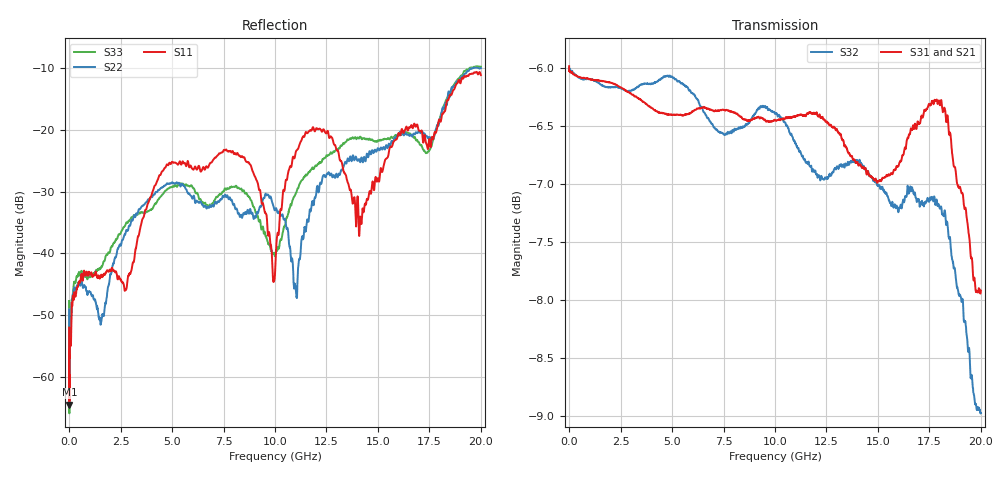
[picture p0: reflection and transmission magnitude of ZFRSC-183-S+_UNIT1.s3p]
!Mini-Circuits Laboratory
!S-Parameters
!Model: ZFRSC-183-S+
!Run/Lot/Date Code: F89730/NA/1038
!Fixture/SN/Due: NOT REQUIRED
!Connection: PORT 1 - SUM, PORT 2 - 1, PORT 3 - 2.
!Tested By: JIAN CHEN
!UNIT S/N: 1
!Agilent Technologies,N5230A,MY45001447,A.07.50.63
!Agilent N5230A: A.07.50.63
!Date: Wednesday, April 06, 2011 14:43:44
!Correction: S11(Full 3 Port(1,2,3))
!S12(Full 3 Port(1,2,3))
!S13(Full 3 Port(1,2,3))
!S21(Full 3 Port(1,2,3))
!S22(Full 3 Port(1,2,3))
!S23(Full 3 Port(1,2,3))
!S31(Full 3 Port(1,2,3))
!S32(Full 3 Port(1,2,3))
!S33(Full 3 Port(1,2,3))
!S3P File: Measurements: <S11,S12,S13>,
!<S21,S22,S23>,
!<S31,S32,S33>:
# Hz S  dB  R 50
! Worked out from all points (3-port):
!   2097 points, 300 kHz to 20 GHz, reference 50 ohm
!   strongest paths, dB at 300 kHz, 4.28 GHz, 9.52 GHz, 14.76 GHz, 20 GHz:
!     S31: -6.0, -6.4, -6.4, -6.9, -7.9
!     S21: -6.0, -6.3, -6.4, -7.0, -8.1
!     S32: -6.0, -6.1, -6.3, -7.0, -9.0
!   lowest |S11| = -64.6 dB at 13 MHz (marker M1), VSWR 1.00, Z = 50 + j0.0587 ohm
!   |S11| at or under -10 dB: start of sweep to end of sweep
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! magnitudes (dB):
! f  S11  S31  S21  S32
! 300 kHz  -52.1  -6.0  -6.0  -6.0
! 13 MHz  -64.6  -6.0  -6.0  -6.0
! 410 MHz  -45.5  -6.1  -6.1  -6.1
! 4.81 GHz  -25.7  -6.4  -6.4  -6.1
! 8.47 GHz  -24.5  -6.4  -6.4  -6.5
! 10.01 GHz  -42.8  -6.4  -6.4  -6.4
! 11 GHz  -23.7  -6.4  -6.4  -6.7
! 11.55 GHz  -20.6  -6.4  -6.4  -6.8
! 14.15 GHz  -34.2  -6.8  -7.0  -6.8
! 20 GHz  -11.1  -7.9  -8.1  -9.0
